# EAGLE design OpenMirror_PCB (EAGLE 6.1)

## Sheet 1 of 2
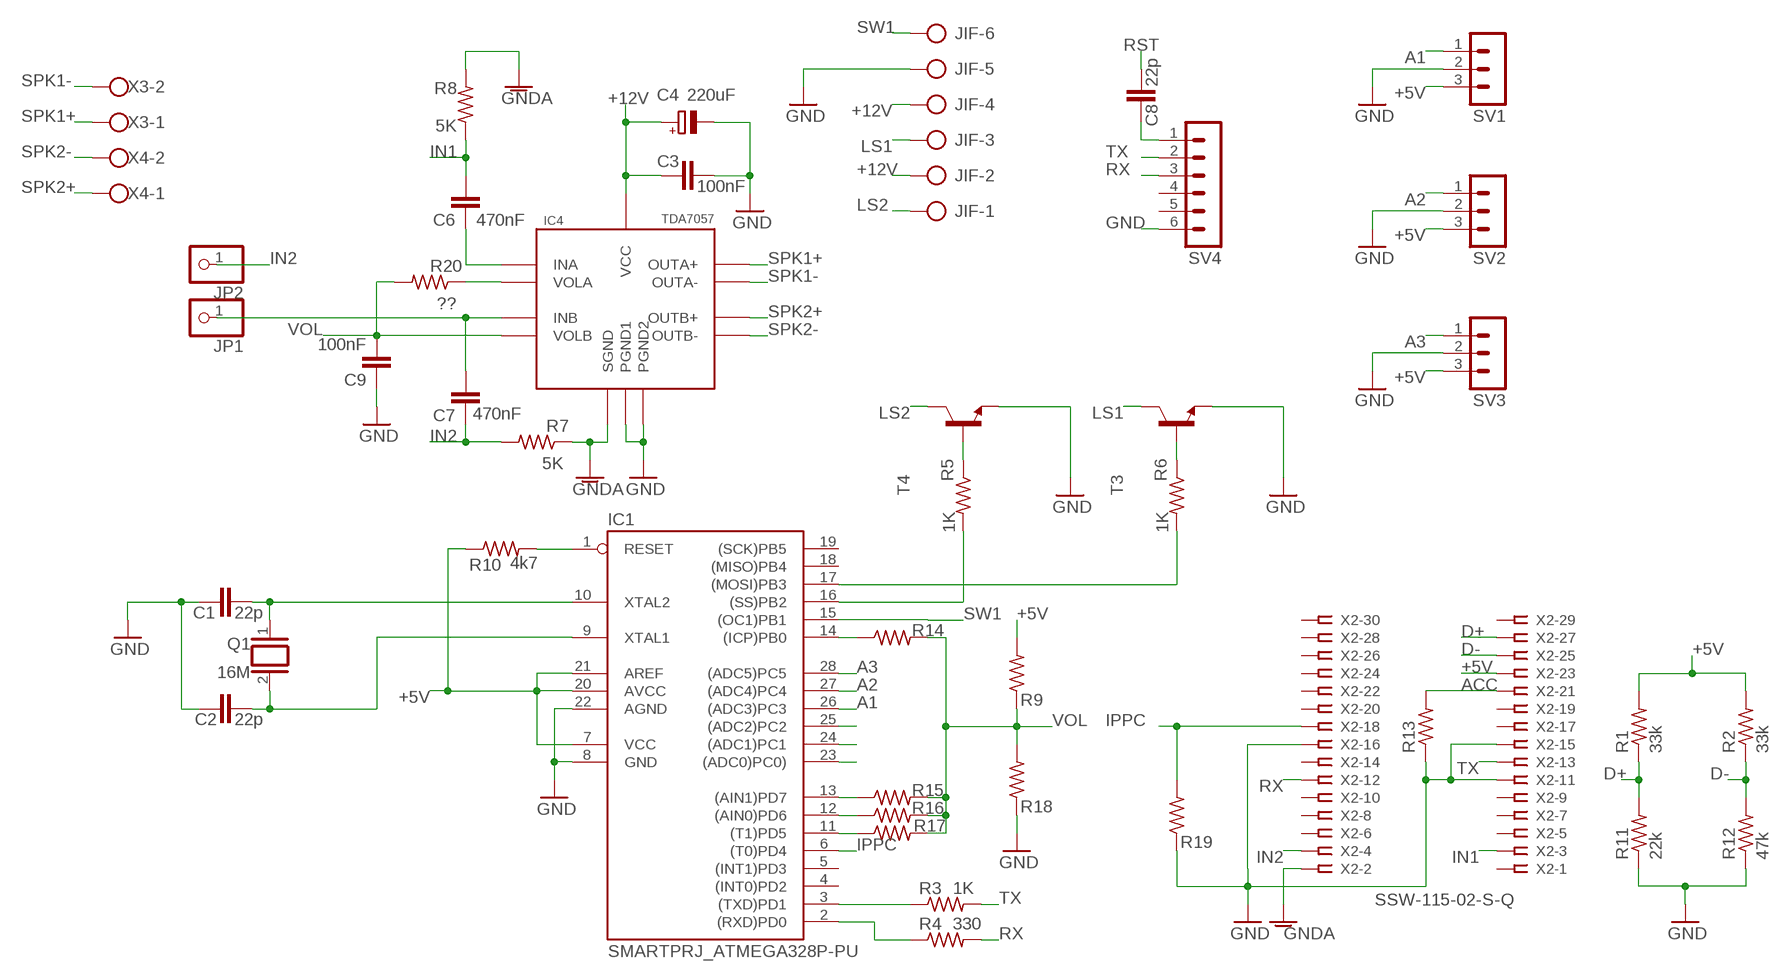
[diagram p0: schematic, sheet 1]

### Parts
C1  22p  C-EU050-024X044  [C050-024X044]
C2  22p  C-EU050-024X044  [C050-024X044]
C3  100nF  C-EU025-025X050  [C025-025X050]
C4  220uF  CPOL-EUE2.5-6  [E2,5-6]
C6  470nF  C-EU050-025X075  [C050-025X075]
C7  470nF  C-EU050-025X075  [C050-025X075]
C8  22p  C-EU050-024X044  [C050-024X044]
C9  100nF  C-EU050-025X075  [C050-025X075]
IC1  SMARTPRJ_ATMEGA328P-PU  [SMARTPRJ_DIL28-3]
IC4  TDA7057  [TDA7057]
JIF  W237-6  [W237-6]
JP1  PINHD-1X1  [1X01]
JP2  PINHD-1X1  [1X01]
Q1  16M  SMARTPRJ_XTAL/S  [SMARTPRJ_QS]
R1  33k  R-US_0207/10  [0207/10]
R2  33k  R-US_0207/10  [0207/10]
R3  1K  R-US_0207/10  [0207/10]
R4  330  R-US_0207/10  [0207/10]
R5  1K  R-US_0207/10  [0207/10]
R6  1K  R-US_0207/10  [0207/10]
R7  5K  R-US_0207/10  [0207/10]
R8  5K  R-US_0207/10  [0207/10]
R9  1k8  R-US_0207/10  [0207/10]
R10  4k7  R-US_0207/15  [0207/15]
R11  22k  R-US_0207/10  [0207/10]
R12  47k  R-US_0207/10  [0207/10]
R13  R-US_0207/10  [0207/10]
R14  1K  R-US_0207/10  [0207/10]
R15  2k2  R-US_0207/10  [0207/10]
R16  3k9  R-US_0207/10  [0207/10]
R17  6k8  R-US_0207/10  [0207/10]
R18  82  R-US_0207/10  [0207/10]
R19  10k  R-US_0207/10  [0207/10]
R20  ??  R-US_0207/2V  [0207/2V]
SV1  MA03-1  [MA03-1]
SV2  MA03-1  [MA03-1]
SV3  MA03-1  [MA03-1]
SV4  MA06-1  [MA06-1]
T3  2N4124-NPN-TO92-CBE  [TO92-CBE]
T4  2N4124-NPN-TO92-CBE  [TO92-CBE]
X2  SSW-115-02-S-Q  [SSW-115-02-S-Q]
X3  W237-102  [W237-102]
X4  W237-102  [W237-102]

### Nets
+5V: IC1.7(VCC) IC1.20(AVCC) IC1.21(AREF) R1.2 R2.2 R9.2 R10.1 SV1.3 SV2.3 SV3.3 X2.23 ; also sheet 2
+12V: C3.1 C4.+ IC4.VCC JIF.2 JIF.4 ; also sheet 2
A1: IC1.26((ADC3)PC3) SV1.1
A2: IC1.27((ADC4)PC4) SV2.1
A3: IC1.28((ADC5)PC5) SV3.1
ACC: R13.2 X2.21
D+: R1.1 R11.2 X2.27
D-: R2.1 R12.2 X2.25
GND: C1.2 C2.2 C3.2 C4.- C9.1 IC1.8(GND) IC1.22(AGND) IC4.PGND1 IC4.PGND2 JIF.5 R11.1 R12.1 R13.1 R18.1 R19.1 SV1.2 SV2.2 SV3.2 SV4.6 T3.E T4.E X2.11 X2.15 X2.16 ; also sheet 2
GNDA: IC4.SGND R7.1 R8.2 X2.2
IN1: C6.2 R8.1 X2.3
IN2: C7.1 JP2.1 R7.2 X2.4
IPPC: IC1.6((T0)PD4) R19.2 X2.18
LS1: JIF.3 T3.C
LS2: JIF.1 T4.C
N$1: IC1.14((ICP)PB0) R14.1
N$2: C1.1 IC1.10(XTAL2) Q1.1
N$3: C2.1 IC1.9(XTAL1) Q1.2
N$4: IC1.13((AIN1)PD7) R15.1
N$5: IC1.3((TXD)PD1) R3.1
N$6: IC1.2((RXD)PD0) R4.1
N$7: R5.1 T4.B
N$8: R6.1 T3.B
N$9: IC1.12((AIN0)PD6) R16.1
N$10: IC1.11((T1)PD5) R17.1
N$11: IC1.17((MOSI)PB3) R6.2
N$12: IC1.16((SS)PB2) R5.2
N$16: C8.2 SV4.1
N$17: IC4.VOLA R20.1
N$18: C6.1 IC4.INA
N$19: C7.2 IC4.INB JP1.1
N$20: IC1.25((ADC2)PC2)
N$21: IC1.24((ADC1)PC1)
N$22: IC1.23((ADC0)PC0))
RST: C8.1 IC1.1(RESET) R10.2
RX: R4.2 SV4.3 X2.12
SPK1+: IC4.OUTA+ X3.1
SPK1-: IC4.OUTA- X3.2
SPK2+: IC4.OUTB+ X4.1
SPK2-: IC4.OUTB- X4.2
SW1: IC1.15((OC1)PB1) JIF.6
TX: R3.2 SV4.2 X2.13
VOL: C9.2 IC4.VOLB R9.1 R14.2 R15.2 R16.2 R17.2 R18.2 R20.2
Unconnected: IC1.4((INT0)PD2) IC1.5((INT1)PD3) IC1.18((MISO)PB4) IC1.19((SCK)PB5) SV4.4 SV4.5 X2.1 X2.5 X2.6 X2.7 X2.8 X2.9 X2.10 X2.14 X2.17 X2.19 X2.20 X2.22 X2.24 X2.26 X2.28 X2.29 X2.30

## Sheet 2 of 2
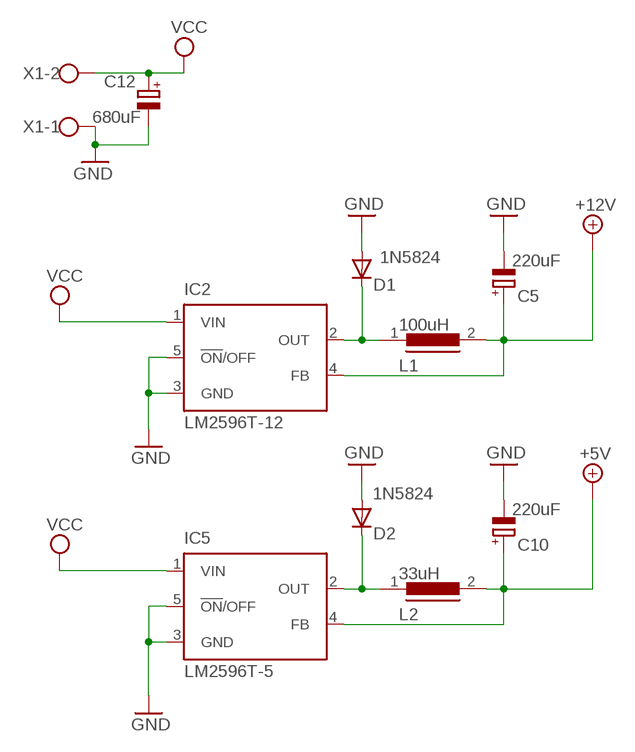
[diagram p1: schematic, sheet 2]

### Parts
C5  220uF  CPOL-EUE3.5-10  [E3,5-10]
C10  220uF  CPOL-EUE3.5-10  [E3,5-10]
C12  680uF  CPOL-EUE3.5-10  [E3,5-10]
D1  1N5059  [DO204-10]
D2  1N5059  [DO204-10]
IC2  LM2596T-12  LM2596T  [T05D]
IC5  LM2596T-5  LM2596T  [T05D]
L1  100uH  SFT840D  [SFT840D]
L2  33uH  SFT840D  [SFT840D]
X1  W237-102  [W237-102]

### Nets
+5V: C10.+ IC5.4(FB) L2.2 ; also sheet 1
+12V: C5.+ IC2.4(FB) L1.2 ; also sheet 1
GND: C5.- C10.- C12.- D1.A D2.A IC2.3(GND) IC2.5(!ON!/OFF) IC5.3(GND) IC5.5(!ON!/OFF) X1.1 ; also sheet 1
N$13: D1.C IC2.2(OUT) L1.1
N$15: D2.C IC5.2(OUT) L2.1
VCC: C12.+ IC2.1(VIN) IC5.1(VIN) X1.2

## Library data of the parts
C1 C2 C6-C8 = rcl:C-EU: CAPACITOR, European symbol
C3 C9 = resistor:C-EU: CAPACITOR, European symbol
C4 C5 C10 C12 = rcl:CPOL-EU: POLARIZED CAPACITOR, European symbol
D1 D2 = diode:1N5059: DIODE; 1N5824: 1N5824
IC1 = arduino_Uno_Rev3-02-TH:SMARTPRJ_ATMEGA328P-: MICROCONTROLLER 4 Kbytes FLASH 128 bytes SRAM 256 bytes EEPROM UART 6-channel 10 bit ADC
IC2 IC5 = national-semiconductor:LM2596: SIMPLE SWITCHER® Power Converter 150 kHz 3A Step-Down Voltage Regulator Source: http://www.national.com/ds/LM/LM2596.pdf; MPN: LM2596T-ADJ/LF02; OC_FARNELL: 9494162; OC_NEWARK: 65K5910
IC4 = TDA7057:TDA7057
JIF = con-wago-500:W237-6: WAGO SCREW CLAMP; OC_FARNELL: unknown; OC_NEWARK: unknown
JP1 JP2 = pinhead:PINHD-1X1: PIN HEADER
L1 L2 = inductors:SFT840D: INDUCTOR
Q1 = arduino_Uno_Rev3-02-TH:SMARTPRJ_XTAL/S: CRYSTAL
R1-R20 = rcl:R-US_: RESISTOR, American symbol
SV1-SV3 = con-lstb:MA03-1: PIN HEADER; OC_FARNELL: unknown; OC_NEWARK: unknown
SV4 = con-lstb:MA06-1: PIN HEADER; OC_FARNELL: unknown; OC_NEWARK: unknown
T3 T4 = transistor:*-NPN-: NPN Transistror BF959 corrected 2008.03.06
X1 X3 X4 = con-wago-500:W237-102: WAGO SCREW CLAMP; MPN: 237-102; OC_FARNELL: unknown; OC_NEWARK: 70K9898
X2 = con-samtec:SSW-115-02-S-Q: THROUGH-HOLE .025" SQ POST SOCKET Source: Samtec SSW.pdf; MPN: SSW-115-02-S-Q; OC_FARNELL: unknown; OC_NEWARK: 82P6863

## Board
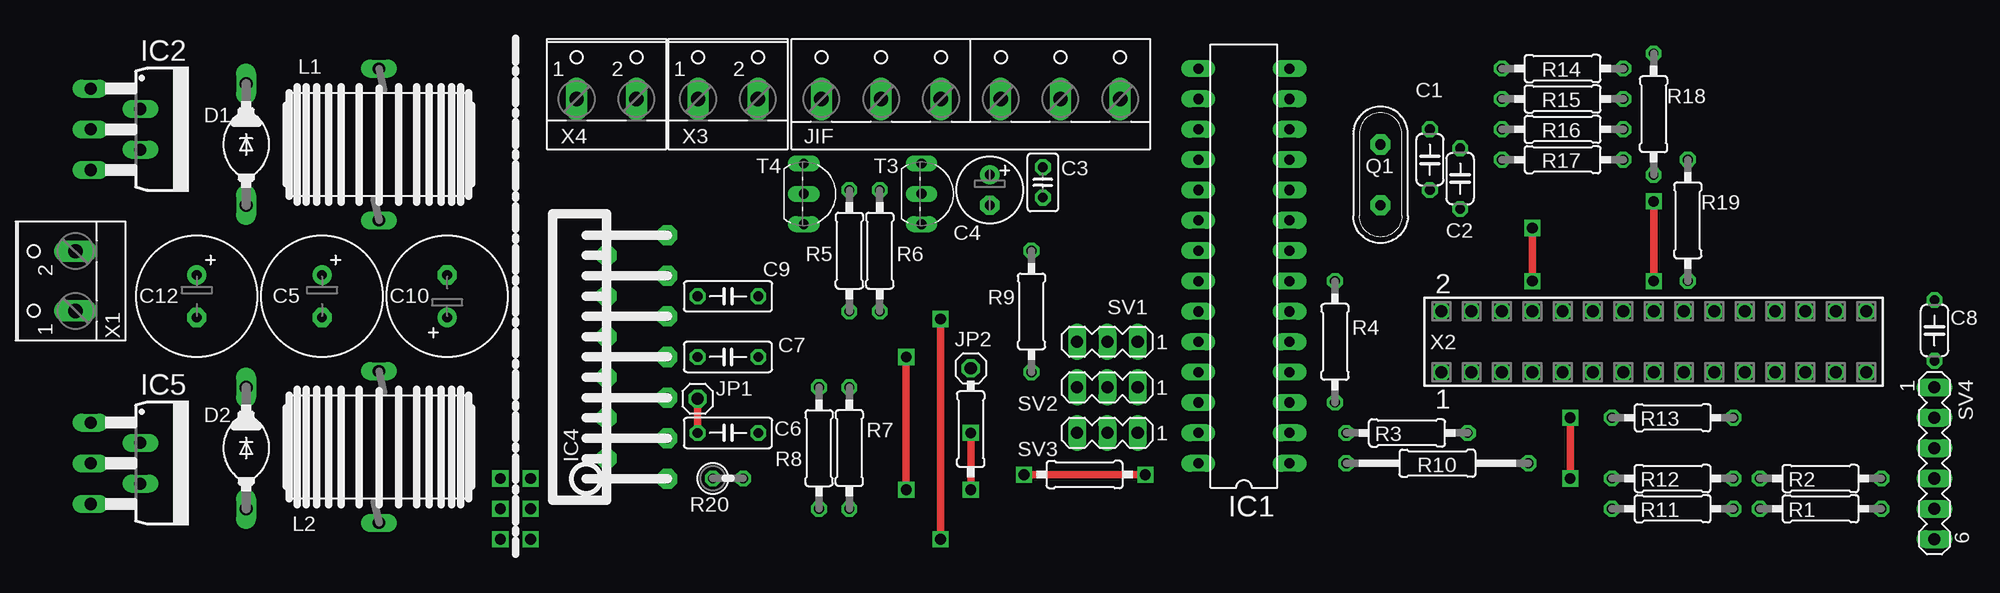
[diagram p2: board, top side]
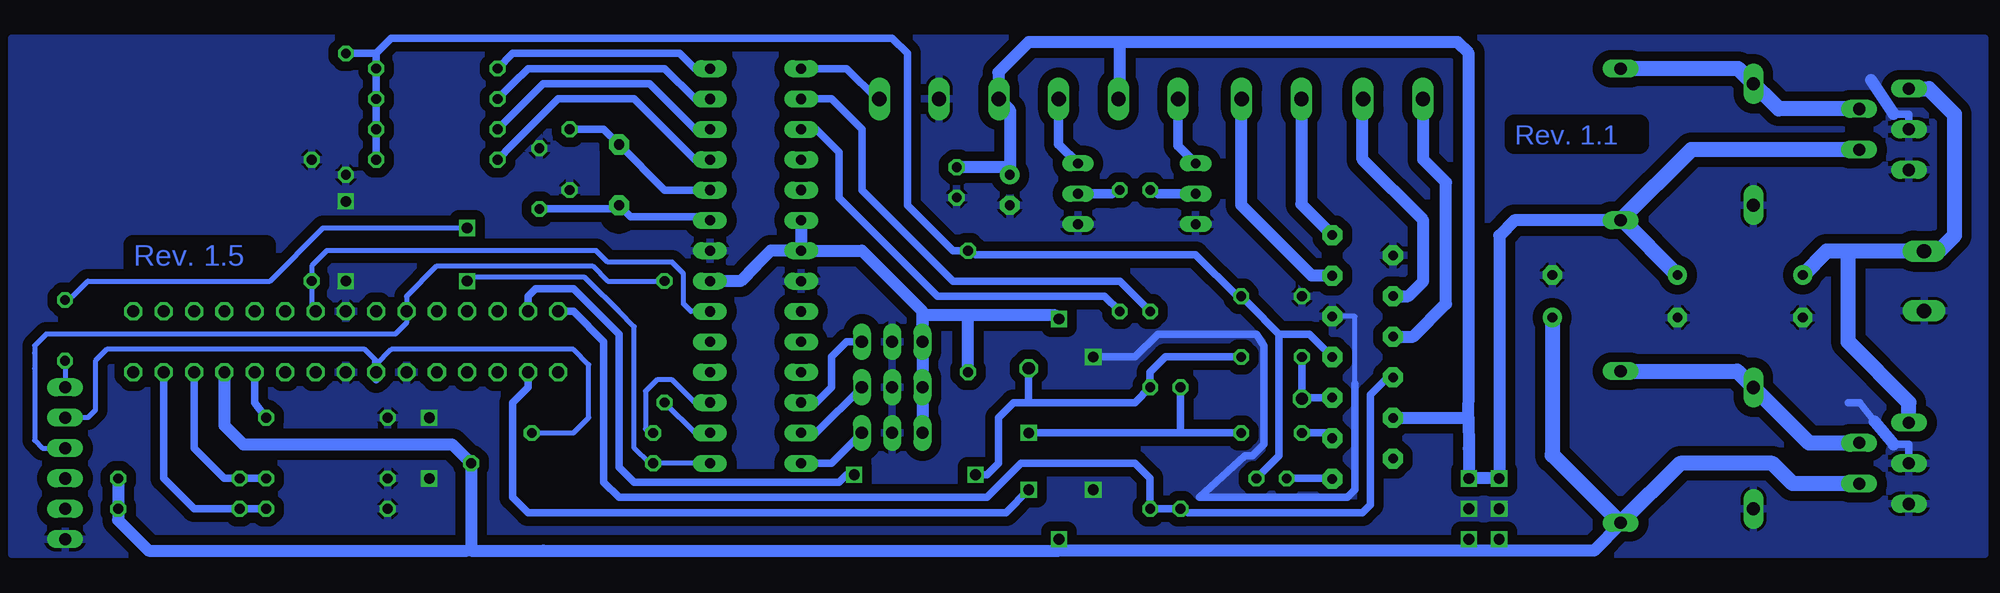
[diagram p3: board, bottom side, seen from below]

No outline drawn. Coordinates in mm, seen from the top.
Copper layers (1*16): Top 0.035mm / dielectric 1.5mm / Bottom 0.035mm
Design rules: minimum track width 10mil, minimum drill 24mil, track to track 8mil, track to pad 8mil, pad to pad 8mil, via to via 8mil, smd to smd 8mil, copper to edge 40mil, drill to drill 8mil, minimum pad ring 10mil, minimum via ring 8mil, stop-mask expansion 4mil, vias tented up to drill 0mil, thermal gap 10mil

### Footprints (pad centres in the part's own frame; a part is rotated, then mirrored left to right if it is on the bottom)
C050-024X044 = drill 0.813 octagon: 1 -2.54,0; 2 2.54,0
C025-025X050 = drill 0.813 octagon: 1 -1.27,0; 2 1.27,0
E2,5-6 = drill 0.813 pad 1.6: + -1.27,0 | drill 0.813 pad 1.6 octagon: - 1.27,0
E3,5-10 = drill 0.813 pad 1.6: + -1.778,0 | drill 0.813 pad 1.6 octagon: - 1.778,0
C050-025X075 = drill 0.813 octagon: 1 -2.54,0; 2 2.54,0
DO204-10 = drill 1.118 long: A 5.08,0; C -5.08,0
SMARTPRJ_DIL28-3 = drill 0.85 pad 1.422 long: 1 -16.51,-3.81; 2 -13.97,-3.81; 3 -11.43,-3.81; 4 -8.89,-3.81; 5 -6.35,-3.81; 6 -3.81,-3.81; 7 -1.27,-3.81; 8 1.27,-3.81; 9 3.81,-3.81; 10 6.35,-3.81; 11 8.89,-3.81; 12 11.43,-3.81; 13 13.97,-3.81; 14 16.51,-3.81; 15 16.51,3.81; 16 13.97,3.81; 17 11.43,3.81; 18 8.89,3.81; 19 6.35,3.81; 20 3.81,3.81; 21 1.27,3.81; 22 -1.27,3.81; 23 -3.81,3.81; 24 -6.35,3.81; 25 -8.89,3.81; 26 -11.43,3.81; 27 -13.97,3.81; 28 -16.51,3.81
T05D = drill 1.016 long: 1 -3.404,-5.08; 2 -1.702,-0.914; 3 0,-5.08; 4 1.702,-0.914; 5 3.404,-5.08
TDA7057 = drill 0.8 pad 1.676 octagon: INA 6.8,5.08; INB 3.4,5.08; NC1 8.5,0; OUTA+ -10.2,5.08; OUTA- -6.8,5.08; OUTB+ -1.7,0; OUTB- -5.1,0; PGND1 -8.5,0; PGND2 -3.4,5.08; SGND 1.7,0; VCC 5.1,0; VOLA 10.2,5.08; VOLB 0,5.08
W237-6 = drill 1.194 long: 1 -12.5,-1.27; 2 -7.5,-1.27; 3 -2.5,-1.27; 4 2.5,-1.27; 5 7.5,-1.27; 6 12.5,-1.27
1X01 = drill 1.016 octagon: 1 0,0
SFT840D = drill 1.016 long: 1 -6.35,0; 2 6.35,0
SMARTPRJ_QS = drill 0.85 pad 1.676 octagon: 1 -2.54,0; 2 2.54,0
0207/10 = drill 0.813 octagon: 1 -5.08,0; 2 5.08,0
0207/15 = drill 0.813 octagon: 1 -7.62,0; 2 7.62,0
0207/2V = drill 0.813 octagon: 1 -1.27,0; 2 1.27,0
MA03-1 = drill 1.016 long: 1 -2.54,0; 2 0,0; 3 2.54,0
MA06-1 = drill 1.016 long: 1 -6.35,0; 2 -3.81,0; 3 -1.27,0; 4 1.27,0; 5 3.81,0; 6 6.35,0
TO92-CBE = drill 0.813 long: B 0,0; C -2.54,0; E 2.54,0
W237-102 = drill 1.194 long: 1 -2.5,-1.27; 2 2.5,-1.27
SSW-115-02-S-Q = drill 1 pad 1.5 octagon: 1 -17.78,-2.54; 2 -17.78,2.54; 3 -15.24,-2.54; 4 -15.24,2.54; 5 -12.7,-2.54; 6 -12.7,2.54; 7 -10.16,-2.54; 8 -10.16,2.54; 9 -7.62,-2.54; 10 -7.62,2.54; 11 -5.08,-2.54; 12 -5.08,2.54; 13 -2.54,-2.54; 14 -2.54,2.54; 15 0,-2.54; 16 0,2.54; 17 2.54,-2.54; 18 2.54,2.54; 19 5.08,-2.54; 20 5.08,2.54; 21 7.62,-2.54; 22 7.62,2.54; 23 10.16,-2.54; 24 10.16,2.54; 25 12.7,-2.54; 26 12.7,2.54; 27 15.24,-2.54; 28 15.24,2.54; 29 17.78,-2.54; 30 17.78,2.54

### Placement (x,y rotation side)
C1  118.43,33.02 270 top
C2  120.97,31.43 90 top
C3  86.04,31.11 270 top
C4  81.6,30.48 270 top
C5  25.72,21.59 270 top
C6  59.69,10.16 0 top
C7  59.69,16.51 180 top
C8  160.66,18.73 270 top
C9  59.69,21.59 0 top
C10  36.2,21.59 90 top
C12  15.24,21.59 270 top
D1  19.37,34.29 270 top
D2  19.37,8.89 270 top
IC1  102.87,24.13 90 top
IC2  11.43,35.56 270 top
IC4  49.53,16.51 270 top
IC5  11.43,7.62 270 top
JIF  80.01,39.37 0 top
JP1  57.15,13.02 0 top
JP2  80.01,15.56 0 top
L1  30.48,34.29 270 top
L2  30.48,8.98 270 top
Q1  114.3,31.75 270 top
R1  151.13,3.81 0 top
R2  151.13,6.35 0 top
R3  116.52,10.16 0 top
R4  110.49,17.78 90 top
R5  69.85,25.4 270 top
R6  72.39,25.4 270 top
R7  69.85,8.89 90 top
R8  67.31,8.89 270 top
R9  85.09,20.32 270 top
R10  119.06,7.62 180 top
R11  138.75,3.81 0 top
R12  138.75,6.35 0 top
R13  138.75,11.43 0 top
R14  129.54,40.64 0 top
R15  129.54,38.1 0 top
R16  129.54,35.56 0 top
R17  129.54,33.02 0 top
R18  137.16,36.83 90 top
R19  140.02,27.94 270 top
R20  59.69,6.35 0 top
SV1  91.44,17.78 180 top
SV2  91.44,13.97 180 top
SV3  91.44,10.16 180 top
SV4  160.66,7.62 270 top
T3  75.88,30.16 270 top
T4  66.04,30.16 270 top
U$1  [RCL_0207/10]  80.01,10.48 90 top
U$2  [RCL_0207/10]  89.53,6.67 180 top
X1  3.81,22.86 90 top
X2  137.16,17.78 0 top
X3  59.69,39.37 0 top
X4  49.53,39.37 0 top

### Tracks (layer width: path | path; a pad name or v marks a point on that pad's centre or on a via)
+5V  (via drill 0.9)
  Top 0.61: v77.47,19.68 v77.47,1.27
  Bottom 0.61: R1.2 R2.2 | 36.2,8.26 30.48,2.54
  Bottom 0.813: 126.68,0.32 120.65,0.32 | 127,0.32 126.68,0.32 | 126.68,0.32 124.46,0.32 126.68,0.32 | 36.2,8.35 C10.+
  Bottom 1.016: IC1.20 IC1.21 | IC1.21 101.6,25.4 102.87,24.13 104.14,22.86 IC1.7 | IC1.21 93.98,25.4 88.9,20.32 | 88.9,20.32 SV1.3 | SV1.3 SV2.3 SV3.3 | 77.47,0.32 120.65,0.32 126.68,0.32 R10.1 128.27,9.21 145.73,9.21 147.32,10.79 X2.23 | 77.47,0.32 v77.47,1.27 | v77.47,19.68 77.79,20 85.09,20 | 85.09,20 88.9,20 SV1.3 | SV1.3 88.9,20.32 | 88.9,20.32 SV1.3 | R2.2 156.21,2.86 153.67,0.32 127,0.32 | 30.48,2.54 32.7,0.32 40.64,0.32 | 40.64,0.32 43.18,0.32 | 43.18,0.32 77.47,0.32 | v43.18,1.27 43.18,0.32 | v40.64,1.27 40.64,0.32 | R9.2 85.09,20
  Bottom 1.27: IC5.4 16.08,5.92 17.78,7.62 25.49,7.62 L2.2 36.2,8.35 | C10.+ 36.2,8.26
+12V  (via drill 0.9)
  Bottom 0.406: JIF.2 72.39,38.1
  Bottom 0.813: 30.29,27.94 L1.2
  Bottom 1.016: 82.55,38.14 82.55,40.32 80.01,42.86 72.39,42.86 | L1.2 39.37,27.94 40.64,26.67 v40.64,6.35 v43.18,6.35 43.18,8.85 43.2,11.41 | 72.39,42.86 44.13,42.86 43.18,41.91 43.18,13.97 43.2,11.41 | C3.1 81.6,32.38 C4.+ 81.6,37.19 82.55,38.14 | IC4.VCC 43.2,11.41 | 72.39,38.1 72.39,42.86 | 82.55,38.14 82.51,38.14 JIF.4
  Bottom 1.27: C5.+ 30.29,27.94 | IC2.4 24.56,33.86 L1.2
A1
  Bottom 0.61: SV1.1 95.25,17.78 96.52,16.51 96.52,13.97 97.79,12.7 IC1.26
A2
  Bottom 0.61: SV2.1 97.79,10.16 IC1.27
A3
  Bottom 0.61: SV3.1 96.52,7.62 IC1.28
ACC
  Bottom 0.61: X2.21 144.78,13.97 144.78,12.7 R13.2
D+
  Bottom 0.61: X2.27 152.4,6.35 149.86,3.81 R1.1 R11.2
D-
  Bottom 0.61: R12.2 R2.1 147.32,6.35 149.86,8.89 X2.25
GND  (via drill 0.9)
  Top 0.61: v74.61,16.51 v74.61,5.4 | v130.18,11.43 v130.18,6.35 | v137.16,22.86 v137.16,29.53
  Bottom 0.406: 52.7,14.29 52.7,19.91 IC4.PGND2
  Bottom 0.61: v74.61,16.51 71.12,16.51 69.22,18.41 60.96,18.41 60.33,17.46 60.33,9.21 60.96,8.57 61.28,8.26 61.91,8.26 65.72,4.76 53.34,4.76 52.7,5.4 52.7,14.29 | 11.43,12.7 10.48,12.7 9.21,11.11 | 7.62,9.21 6.35,9.21 IC5.3 | 7.62,36.83 6.35,36.83 IC2.3
  Bottom 1.016: 9.21,11.11 7.62,9.21 | 9.53,39.69 7.62,36.83
  other vias: 43.18,3.81 40.64,3.81
  pour Bottom (isolate 0.813): 0,43.18 165.1,43.18 165.1,0 0,0
GNDA
  Bottom 0.61: IC4.SGND 49.96,14.81 51.44,13.34 51.44,4.13 52.07,3.49 66.67,3.49 R8.2 | R8.2 R7.1 | R7.1 R8.2 | X2.2 118.11,20.32 115.57,17.78 115.57,16.51 115.57,13.97 115.57,6.03 114.3,4.76 109.22,4.76 83.5,4.76 80.64,7.62 71.12,7.62 69.85,6.35 R7.1 | R7.1 R8.2
IN1  (via drill 0.9)
  Top 0.61: v80.01,10.16 v80.01,5.4
  Bottom 0.61: v80.01,5.4 81.92,3.49 83.82,3.49 115.57,3.49 116.84,3.49 121.92,3.49 123.19,4.76 123.19,12.7 121.92,13.97 X2.3 | C6.2 63.5,10.16 67.31,10.16 | 67.31,10.16 R8.1 67.31,10.16 | 67.31,10.16 v80.01,10.16
IN2  (via drill 0.9)
  Top 0.61: v94.61,6.67 v84.45,6.67
  Bottom 0.61: X2.4 121.92,21.59 121.28,22.23 118.11,22.23 114.3,18.41 114.3,7.3 113.03,6.03 97.79,6.03 95.89,6.03 95.25,6.67 v94.61,6.67 | C7.1 64.77,16.51 67.31,16.51 68.58,16.51 69.85,15.24 R7.2 71.12,12.7 80.01,12.7 | 80.01,12.7 81.28,12.7 82.55,11.43 82.55,7.62 83.5,6.67 84.14,6.67 v84.45,6.67 | JP2.1 80.01,12.7
IPPC
  Bottom 0.406: X2.18 140.02,20.64 R19.2 140.02,24.13 138.75,25.4 136.21,25.4 130.49,25.4 124.46,25.4 116.2,25.4 115.25,24.45 111.12,24.45 109.86,24.45 108.9,23.5 108.9,20.95 108.27,20.32 IC1.6
LS1
  Bottom 0.813: JIF.3 77.51,34.33 T3.C
LS2
  Bottom 0.813: JIF.1 67.51,34.17 T4.C
N$1
  Bottom 0.61: IC1.14 107.95,40.64 109.22,41.91 123.19,41.91 R14.1
N$2
  Bottom 0.61: Q1.1 114.62,34.29 Q1.1 | Q1.1 115.57,35.56 C1.1 | IC1.10 107.95,30.48 110.49,30.48 Q1.1
N$3
  Bottom 0.61: C2.1 114.62,28.89 Q1.2 113.35,28.26 107,28.26 IC1.9
N$4
  Bottom 0.61: IC1.13 107.95,38.1 110.49,40.64 121.92,40.64 123.19,39.37 R15.1
N$5
  Bottom 0.406: IC1.3 107.95,12.7 109.86,14.61 111.12,14.61 112.08,13.65 112.08,10.48 111.76,10.16 R3.1
N$6
  Bottom 0.406: R4.1 107.95,10.16 IC1.2
N$7
  Bottom 0.813: T4.B 69.22,30.16 R5.1
N$8
  Bottom 0.813: R6.1 73.03,30.16 T3.B
N$9
  Bottom 0.61: IC1.12 107.95,35.56 111.76,39.37 120.65,39.37 123.19,36.83 R16.1
N$10
  Bottom 0.61: IC1.11 107.95,33.02 113.03,38.1 115.57,38.1 119.38,38.1 123.19,34.29 R17.1
N$11
  Bottom 0.61: R6.2 73.66,21.59 87.63,21.59 95.89,29.84 95.89,33.66 97.79,35.56 IC1.17
N$12
  Bottom 0.61: IC1.16 96.52,38.1 93.98,35.56 93.98,30.48 86.36,22.86 72.39,22.86 71.12,21.59 R5.2
N$13
  Bottom 0.813: D1.C 19.84,39.85
  Bottom 1.27: L1.1 20.64,40.64 19.84,39.85 17.26,37.26 IC2.2
N$14
  cutout Bottom (no thermals): 112.71,34.92 112.71,28.57 arc180 115.89,28.26 115.89,34.61 arc180
N$15
  Bottom 1.27: L2.1 20.73,15.33 D2.C 14.72,9.32 IC5.2
N$16
  Bottom 0.406: C8.2 SV4.1
N$17
  Bottom 0.61: R20.1 57.15,6.35 54.61,6.35 IC4.VOLA
N$18
  Top 0.61: 57.15,12.7 C6.1
  Bottom 0.61: IC4.INA 55.11,10.16 C6.1
N$19
  Bottom 0.61: C7.2 JP1.1 57.15,13.11 IC4.INB
RST  (via drill 0.9)
  Top 0.61: v127,22.86 v127,27.3
  Bottom 0.406: IC1.1 R10.2 | 111.76,7.62 113.03,8.89 113.03,19.05 114.3,20.32 116.84,22.86 117.16,23.18 126.68,23.18 v127,22.86 | C8.1 160.02,21.59 158.75,22.86 143.51,22.86 139.06,27.3 v127,27.3
  Bottom 0.61: R10.2 111.76,7.62
RX
  Bottom 0.406: R4.2 111.12,22.86 115.25,22.86 116.52,24.13 123.19,24.13 123.83,24.13 124.46,24.13 129.54,24.13 132.08,21.59 X2.12 132.08,19.37 133.03,18.41 156.53,18.41 160.34,18.41 162.24,18.41 163.19,17.46 | 163.19,17.46 163.19,16.83 | 163.19,17.46 163.19,16.83 | 163.19,16.83 163.19,15.56 163.19,9.53 162.56,8.89 SV4.3
SPK1+
  Bottom 1.016: X3.1 57.19,29.29 IC4.OUTA+
SPK1-
  Bottom 0.61: 62.23,38.06 X3.2
  Bottom 1.016: IC4.OUTA- 56.33,23.31 62.23,29.21 62.23,38.06
SPK2+
  Bottom 1.016: IC4.OUTB+ 47.83,18.21 45.09,20.95 45.09,31.11 46.99,33.02 46.99,36.83 46.99,38.06 X4.1
SPK2-
  Bottom 0.61: 52.07,38.06 X4.2
  Bottom 1.016: IC4.OUTB- 48.24,21.61 46.99,22.86 46.99,27.94 52.07,33.02 52.07,38.06
SW1
  Bottom 0.61: IC1.15 95.25,40.64 92.71,38.1
  Bottom 0.813: 92.71,38.1 JIF.6
TX
  Bottom 0.406: 134.62,14.61 X2.13 134.62,15.88 | 134.62,15.88 134.62,16.19 134.78,16.35 | 134.78,16.35 135.57,17.14 157.16,17.14 158.12,16.19 158.12,12.06 158.75,11.43 160.34,11.43 SV4.2 | R3.2 120.65,10.16 118.11,10.16 116.84,11.43 116.84,15.88 118.11,17.14 133.35,17.14 134.62,15.88 | 134.78,16.35 134.78,15.4
  Bottom 0.61: 134.62,14.61 X2.13 | X2.13 134.62,15.88 | 134.78,15.4 X2.13
VCC
  Bottom 0.813: 3.81,25.4 X1.2
  Bottom 1.27: 3.81,25.4 2.54,26.67 2.54,29.17 2.54,36.83 4.67,38.96 IC2.1 | X1.2 11.43,25.36 | 11.43,25.36 13.25,25.36 C12.+ | IC5.1 6.35,11.43 6.35,12.7 11.43,17.78 11.43,25.36
VOL
  Bottom 0.406: R9.1 86.36,25.4
  Bottom 0.61: R14.2 R15.2 | R15.2 R16.2 | R16.2 R17.2 | R14.2 134.62,41.91 | 134.62,41.91 133.35,43.18 91.44,43.18 90.17,41.91 90.17,35.56 90.17,29.21 86.36,25.4 R9.1 84.45,25.08 67.31,25.08 66.04,25.08 62.55,21.59 C9.2 61.59,20.95 59.05,18.41 | R14.2 R15.2 | R15.2 R16.2 | R16.2 R15.2 | IC4.VOLB 55.88,17.78 56.52,18.41 59.05,18.41 | 59.05,18.41 59.05,13.97 59.05,8.26 R20.2 | R18.2 134.62,41.91

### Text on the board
Bottom: Rev. 1.1 | Rev. 1.5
